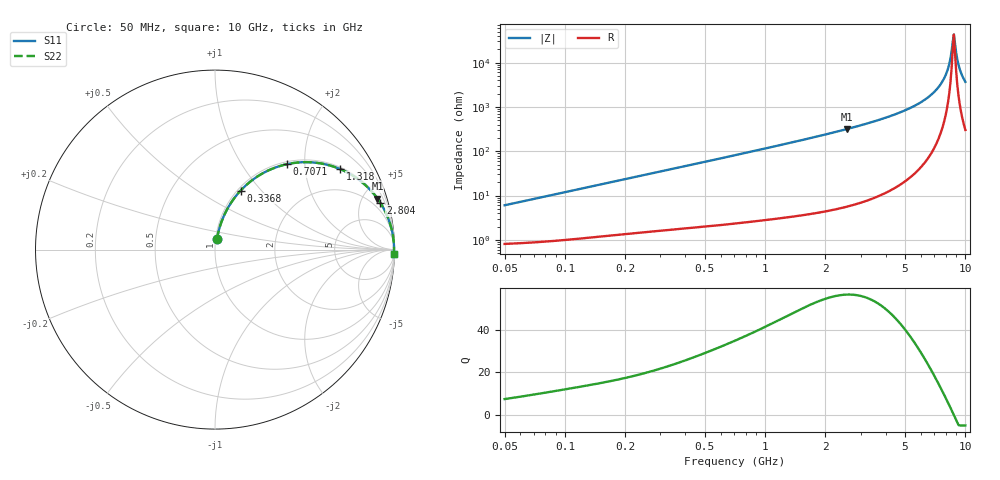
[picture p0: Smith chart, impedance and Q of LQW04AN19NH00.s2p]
!Murata Part Number: LQW04AN19NH00
!These Parameters are Measured in Series Mode Connection
!  o--[Z]--o
!Port1  Port2
!  o-------o
!Freq. Start=50[MHz] Stop=10[GHz], 401[Steps]
# Hz S RI R 50
!Freq.(Hz)	S 11(Real)	S 11(Imag)	S 21(Real)	S 21(Imag)	S 12(Real)	S 12(Imag)	S 22(Real)	S 22(Imag)
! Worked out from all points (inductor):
!   401 points, 50 MHz to 10 GHz, reference 50 ohm
!   read as one part in series: L = 19 nH near 51.34 MHz
!   highest Q = 56.4 at 2.556 GHz (marker M1), where L = 19.7 nH
!   self-resonance near 8.644 GHz
!   S11 on the Smith chart (normalised r, x): 50 MHz: 1.02, +0.12; 336.8 MHz: 1.03, +0.78; 707.1 MHz: 1.05, +1.63; 1.318 GHz: 1.07, +3.06; 2.804 GHz: 1.13, +7.07; 10 GHz: 7, -73
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5e7  0.0115 0.0587  0.9885 -0.0587  0.9885 -0.0587  0.0115 0.0587
1.214486e8  0.0302 0.1377  0.9698 -0.1377  0.9698 -0.1377  0.0302 0.1377
2.949953e8  0.1159 0.2977  0.8841 -0.2977  0.8841 -0.2977  0.1159 0.2977
3.367757e8  0.1425 0.3286  0.8575 -0.3286  0.8575 -0.3286  0.1425 0.3286
7.071068e8  0.4013 0.476  0.5987 -0.476  0.5987 -0.476  0.4013 0.476
1.31782e9  0.6974 0.4488  0.3026 -0.4488  0.3026 -0.4488  0.6974 0.4488
1.717543e9  0.7995 0.3909  0.2005 -0.3909  0.2005 -0.3909  0.7995 0.3909
2.555552e9  0.905 0.2845  0.095 -0.2845  0.095 -0.2845  0.905 0.2845
2.803837e9  0.922 0.2594  0.078 -0.2594  0.078 -0.2594  0.922 0.2594
4.171863e9  0.9707 0.1585  0.0293 -0.1585  0.0293 -0.1585  0.9707 0.1585
5.809576e9  0.9901 0.0841  0.00986 -0.0841  0.00986 -0.0841  0.9901 0.0841
7.181012e9  0.9959 0.04  0.00407 -0.04  0.00407 -0.04  0.9959 0.04
7.672705e9  0.9969 0.0265  0.00311 -0.0265  0.00311 -0.0265  0.9969 0.0265
7.983737e9  0.9973 0.0185  0.00271 -0.0185  0.00271 -0.0185  0.9973 0.0185
8.307378e9  0.9976 0.0105  0.00245 -0.0105  0.00245 -0.0105  0.9976 0.0105
8.530394e9  0.9977 0.00513  0.00235 -0.00513  0.00235 -0.00513  0.9977 0.00513
8.644138e9  0.9977 0.00246  0.00232 -0.00246  0.00232 -0.00246  0.9977 0.00246
8.759398e9  0.9977 -0.000209  0.0023 0.000209  0.0023 0.000209  0.9977 -0.000209
8.876195e9  0.9977 -0.00288  0.0023 0.00288  0.0023 0.00288  0.9977 -0.00288
9.236013e9  0.9976 -0.0109  0.00239 0.0109  0.00239 0.0109  0.9976 -0.0109
9.48396e9  0.9975 -0.0162  0.00252 0.0162  0.00252 0.0162  0.9975 -0.0162
1e10  0.997 -0.0269  0.00295 0.0269  0.00295 0.0269  0.997 -0.0269
